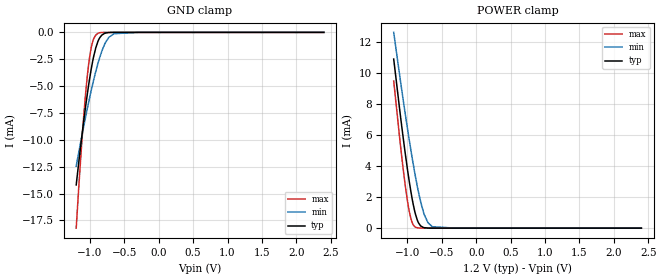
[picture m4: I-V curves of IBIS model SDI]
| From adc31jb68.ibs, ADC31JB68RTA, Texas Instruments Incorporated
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|   Model SDI
[Model]   SDI
Model_type   Input
Vinl = 0.3
Vinh = 0.9
|   typ   min   max
|   (nom PVT)   (slow PVT)   (fast PVT)
C_comp   0.100pF   0.058pF   0.196pF
[Voltage Range]   1.2   1.15   1.25
[Temperature Range]   27   125   -40
[Power Clamp Reference]   1.2   1.15   1.25
[GND Clamp Reference]   0   0   0
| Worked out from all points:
|   GND clamp passes 1 mA (typ) near -0.89 V on its own axis
|   POWER clamp passes 1 mA (typ) near -0.89 V on its own axis
[GND Clamp]
|   Voltage   I(typ)   I(min)   I(max)
-1.2V     -14.19mA   -12.45mA   -18.21mA
-1.16V    -11.95mA   -11.08mA   -14.16mA
-1.099V   -8.68mA    -9.032mA   -8.511mA
-1.063V   -6.893mA   -7.871mA   -5.692mA
-1.034V   -5.562mA   -6.972mA   -3.81mA
-980.4mV  -3.37mA    -5.371mA   -1.383mA
-951.6mV  -2.406mA   -4.571mA   -684.3uA
-915.6mV  -1.444mA   -3.636mA   -244.4uA
-858mV    -499.3uA   -2.325mA   -31.59uA
-782.4mV  -81.98uA   -1.047mA   -932.5nA
-649.2mV  -898.5nA   -124uA     -35.95nA
2.4V      0A         0A         0A
[POWER Clamp]
|   Voltage   I(typ)   I(min)   I(max)
-1.2V     10.91mA    12.64mA    9.501mA
-1.106V   7.403mA    9.642mA    5.527mA
-1.056V   5.625mA    8.09mA     3.592mA
-1.002V   3.856mA    6.489mA    1.814mA
-951.6mV  2.394mA    5.071mA    641.7uA
-922.8mV  1.678mA    4.302mA    270.4uA
-894mV    1.078mA    3.572mA    94.67uA
-840mV    343.8uA    2.331mA    10.69uA
-757.2mV  30.07uA    893.7uA    278.9nA
-703.2mV  5.289uA    358uA      19.36nA
-638.4mV  576.1nA    89.3uA     0A
2.4V      0A         0A         0A
